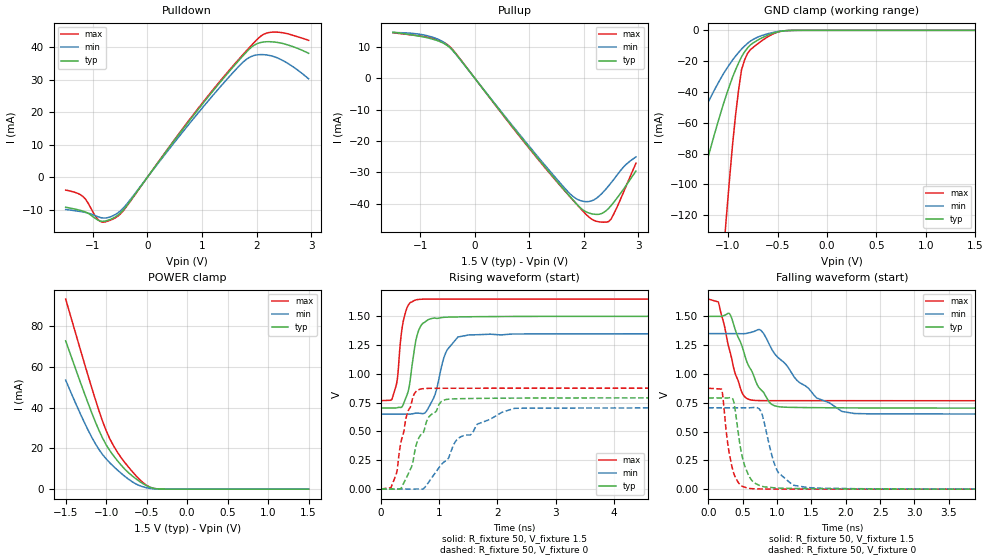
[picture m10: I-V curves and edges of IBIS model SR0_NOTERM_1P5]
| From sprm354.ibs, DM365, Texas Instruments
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|   Model Cell SR0_NOTERM_1P5
|SR0_NOTERM_1P5
[Model]   SR0_NOTERM_1P5
Model_type   I/O
Polarity   Non-Inverting
Enable   Active-Low
Vinl = 0.8V
Vinh = 2V
Cref =  15.0000pF
Rref =  100.0000M
Vref =  0V
Vmeas =  0.75
C_comp   3.047242p   2.257596p   4.009695p
[Model Spec]
Vinl   0.8V   0.8V   0.8V
Vinh   2V   2V   2V
[Temperature Range]   25   125   -40
[Voltage Range]   1.5   1.35   1.65
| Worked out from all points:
|   slope of the pulldown table from 0 to 0.225 V, typ, clamps not added: 43.5 ohm
|   slope of the pullup table from 0 to 0.225 V, typ, clamps not added: 44.5 ohm
|   GND clamp passes 1 mA (typ) near -0.50 V on its own axis
|   POWER clamp passes 1 mA (typ) near -0.46 V on its own axis
|   rising waveform, R_fixture 50, V_fixture 1.5: 20-80 % time 149ps typ, 233ps min, 112ps max; typ from 0.703 V to 1.5 V
|   rising waveform, R_fixture 50, V_fixture 0: 20-80 % time 342ps typ, 724ps min, 210ps max; typ from 0 V to 0.792 V
|   falling waveform, R_fixture 50, V_fixture 1.5: 20-80 % time 348ps typ, 649ps min, 222ps max; typ from 1.5 V to 0.703 V
|   falling waveform, R_fixture 50, V_fixture 0: 20-80 % time 156ps typ, 201ps min, 124ps max; typ from 0.792 V to 0 V
[POWER_clamp]
|   voltage   I(typ)   I(min)   I(max)
-1.5V     72.7mA     53.44mA    93.18mA
-1.318V   52.38mA    36.88mA    68.36mA
-1.182V   37.83mA    25.73mA    50.18mA
-1.091V   29.01mA    19.56mA    38.72mA
-1V       21.75mA    14.84mA    28.68mA
-909.1mV  16.39mA    11.15mA    21.28mA
-818.2mV  11.93mA    7.901mA    15.6mA
-681.8mV  6.623mA    3.713mA    8.833mA
-545.5mV  2.678mA    1.141mA    3.213mA
-454.5mV  887.8uA    343.9uA    858.6uA
-363.6mV  140.3uA    66.33uA    91.97uA
1.5V      4.339nA    108.4nA    952.4pA
[Pulldown]
|   voltage   I(typ)   I(min)   I(max)
-1.5V     -9.235mA   -9.935mA   -3.974mA
-1.182V   -10.44mA   -10.7mA    -5.949mA
-954.5mV  -12.72mA   -11.86mA   -12.01mA
-863.6mV  -13.5mA    -12.42mA   -13.62mA
-590.9mV  -12.24mA   -11.5mA    -12.52mA
-363.6mV  -8.405mA   -7.956mA   -8.569mA
1V        22.28mA    21.15mA    22.64mA
1.818V    38.51mA    36.26mA    38.89mA
2V        40.95mA    37.55mA    42.14mA
2.227V    41.63mA    37.44mA    44.44mA
2.545V    40.77mA    35.25mA    44.16mA
2.955V    38.06mA    30.23mA    42.04mA
[Pullup]
|   voltage   I(typ)   I(min)   I(max)
-1.5V     14.7mA     14.52mA    14.5mA
-863.6mV  12.86mA    13.51mA    13.07mA
-636.4mV  11.64mA    12.11mA    11.96mA
-454.5mV  9.734mA    9.774mA    10.01mA
909.1mV   -20.18mA   -19.79mA   -20.43mA
1.682V    -36.4mA    -35.65mA   -36.52mA
1.909V    -40.82mA   -38.81mA   -40.93mA
2.182V    -43.3mA    -38.76mA   -45.27mA
2.364V    -42.76mA   -36.1mA    -45.85mA
2.5V      -40.54mA   -33.29mA   -44.83mA
2.727V    -35.31mA   -28.29mA   -36.29mA
2.955V    -29.56mA   -25.07mA   -27.07mA
[GND_clamp]
|   voltage   I(typ)   I(min)   I(max)
-1.5V     -154.8mA   -88.21mA   -548.3mA
-1.379V   -125mA     -70.97mA   -438.6mA
-1.045V   -47.59mA   -28.12mA   -144.3mA
-1.015V   -41.63mA   -25.03mA   -120mA
-954.5mV  -30.51mA   -19.31mA   -74.42mA
-924.2mV  -25.71mA   -16.8mA    -55.35mA
-863.6mV  -17.19mA   -12.18mA   -25.62mA
-803mV    -11.46mA   -8.491mA   -15.01mA
-742.4mV  -8.023mA   -5.77mA    -10.9mA
-560.6mV  -2.222mA   -1.606mA   -2.834mA
-409.1mV  -188.4uA   -199.7uA   -167.9uA
1.5V      4.339nA    679.1nA    663.7pA
[Ramp]
| variable   typ   min   max
dV/dt_f   0.494457/0.3522576n   0.440711/0.6626204n  0.5421663/0.2286156n
dV/dt_r  0.4755293/0.3418196n   0.424077/0.7240577n  0.5260539/0.2087291n
R_load = 50
[Rising Waveform]
R_fixture = 50
V_fixture = 1.5
V_fixture_min = 1.35
V_fixture_max = 1.65
|   time   V(typ)   V(min)   V(max)
0s        703.4mV    650.3mV    767.7mV
175.2ps   703.4mV    650.3mV    771.6mV
253.6ps   703.4mV    650.3mV    883.1mV
370.4ps   719.2mV    650.3mV    1.418V
483.2ps   879.8mV    650.1mV    1.606V
588ps     1.256V     658.1mV    1.641V
803.2ps   1.468V     693.1mV    1.65V
1.111ns   1.492V     1.182V     1.65V
1.322ns   1.495V     1.32V      1.65V
5.59ns    1.5V       1.349V     1.65V
[Rising Waveform]
R_fixture = 50
V_fixture = 0
V_fixture_min = 0
V_fixture_max = 0
|   time   V(typ)   V(min)   V(max)
0s        69.34nV    280.7nV    23.27nV
172.8ps   5.752uV    354.3nV    11.77mV
278.4ps   -454.1uV   -384.1nV   158.9mV
344.8ps   6.324mV    1.025uV    406.7mV
558.4ps   258.6mV    -674.3uV   810.1mV
678.4ps   467mV      -933.4uV   867.7mV
1.08ns    772.1mV    233.9mV    875.3mV
1.326ns   784.1mV    439mV      875.5mV
2.294ns   789.6mV    701.2mV    875.8mV
6.759ns   791.6mV    705mV      875.8mV
[Falling Waveform]
R_fixture = 50
V_fixture = 1.5
V_fixture_min = 1.35
V_fixture_max = 1.65
|   time   V(typ)   V(min)   V(max)
0s        1.5V       1.35V      1.65V
148ps     1.5V       1.35V      1.625V
313.6ps   1.52V      1.35V      1.2V
481.6ps   1.258V     1.349V     851.8mV
615.2ps   1.043V     1.36V      775.3mV
764.8ps   863.9mV    1.38V      768.6mV
968ps     723.1mV    1.173V     768.1mV
1.577ns   707.2mV    791.4mV    767.9mV
1.943ns   705.7mV    674.9mV    767.9mV
5.971ns   703.5mV    651.7mV    767.7mV
[Falling Waveform]
R_fixture = 50
V_fixture = 0
V_fixture_min = 0
V_fixture_max = 0
|   time   V(typ)   V(min)   V(max)
0s        791.6mV    706.4mV    875.8mV
200ps     791.6mV    706.4mV    854.6mV
285.6ps   791.5mV    706.4mV    387.8mV
362.4ps   775.9mV    706.4mV    155.2mV
476ps     335.2mV    706.4mV    32.55mV
558.4ps   160.4mV    706.2mV    11.64mV
765.6ps   27.69mV    677mV      1.612mV
996ps     10.19mV    170.1mV    648.8uV
1.232ns   6.143mV    34.67mV    276.2uV
6.133ns   46.86uV    1.351mV    25.02nV
